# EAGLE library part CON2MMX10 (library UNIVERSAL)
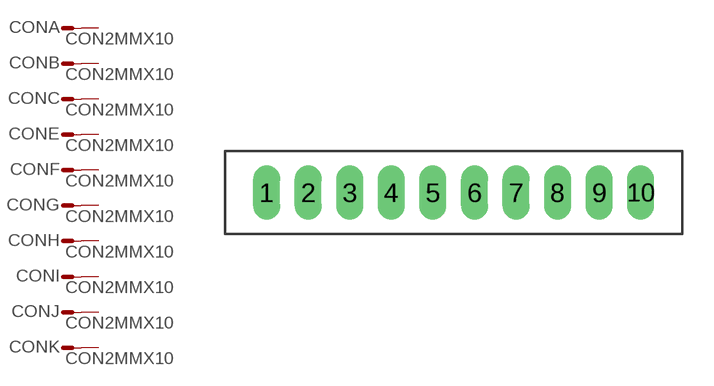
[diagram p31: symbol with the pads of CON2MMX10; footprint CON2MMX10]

Designator prefix CON; gates A=CONPIN B=CONPIN C=CONPIN E=CONPIN F=CONPIN G=CONPIN H=CONPIN I=CONPIN J=CONPIN K=CONPIN

## CON2MMX10  [CON2MMX10]
1  A:S  pas
2  B:S  pas
3  C:S  pas
4  E:S  pas
5  F:S  pas
6  G:S  pas
7  H:S  pas
8  I:S  pas
9  J:S  pas
10  K:S  pas

## Footprint CON2MMX10 (pad centres in mm)
drill 0.8 pad 1.016 long: 1 2,2; 2 4,2; 3 6,2; 4 8,2; 5 10,2; 6 12,2; 7 14,2; 8 16,2; 9 18,2; 10 20,2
